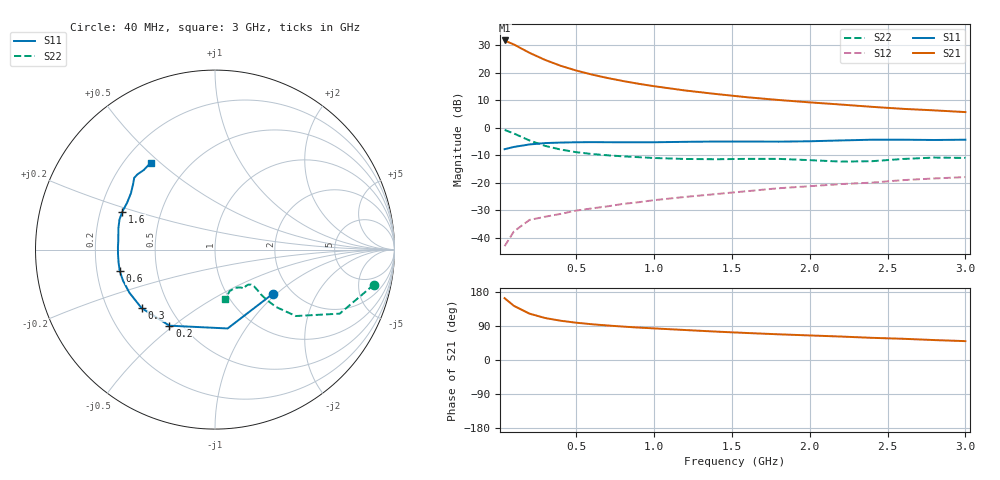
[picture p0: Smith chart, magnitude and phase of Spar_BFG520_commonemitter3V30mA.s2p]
! Filename:  BFG520F.S2P  Version:  2.1
! NXP part #: BFG520  Date: Feb 1992
! Bias condition: Vce=3V, Ic=30mA
! IN LINE PINNING: same data as with cross emitter pinning.
#  MHz  S  MA  R  50
! Freq  S11  S21  S12  S22  !GUM [dB]
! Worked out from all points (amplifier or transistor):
!   21 points, 40 MHz to 3 GHz, reference 50 ohm
!   highest |S21| = 31.7 dB at 40 MHz (marker M1)
!   |S21| within 3 dB of that: start of sweep to 150.3 MHz
!   unconditionally stable (mu >= 1): 627.5 MHz to end of sweep
!   at 300 MHz: K = 0.67, MSG = 28.5 dB, |S12| = -32.4 dB
!   at 1 GHz: K = 1.19, MAG = 18.1 dB, |S12| = -26.4 dB
!   at 3 GHz: K = 1.29, MAG = 8.6 dB, |S12| = -18.0 dB
!   S11 on the Smith chart (normalised r, x): 40 MHz: 1.60, -0.95; 200 MHz: 0.43, -0.48; 300 MHz: 0.35, -0.31; 600 MHz: 0.30, -0.10; 1.6 GHz: 0.29, +0.18; 3 GHz: 0.31, +0.47
40  0.405 -37.6  38.3 163.1  0.007 75.3  0.907 -12.4
100  0.445 -80.9  32.27 142.8  0.013 64.8  0.781 -27.2
200  0.494 -120.9  22.82 122.3  0.021 54.9  0.583 -39.4
300  0.523 -141.4  16.96 110.8  0.024 52.4  0.465 -43.3
400  0.534 -153.3  13.27 103.6  0.027 54.0  0.399 -44.2
500  0.541 -161.4  10.88 98.4  0.031 55.0  0.357 -44.3
600  0.544 -167.4  9.206 94.4  0.034 57.2  0.331 -43.7
700  0.542 -172.3  7.97 91.1  0.037 59.0  0.314 -43.5
800  0.541 -177.1  7.019 88.2  0.041 61.1  0.3 -43.2
900  0.541 178.5  6.255 85.6  0.044 63.2  0.29 -43.4
1000  0.541 174.6  5.65 83.4  0.048 64.8  0.28 -44.1
1200  0.551 167.7  4.721 79.1  0.055 66.4  0.269 -46.6
1400  0.558 162.5  4.07 74.9  0.062 67.7  0.266 -50.1
1600  0.558 157.8  3.553 71.2  0.07 69.7  0.27 -52.3
1800  0.555 152.0  3.172 67.8  0.079 69.5  0.27 -53.4
2000  0.564 146.1  2.871 64.8  0.086 70.9  0.256 -55.5
2200  0.584 141.4  2.622 61.9  0.094 71.0  0.241 -61.8
2400  0.602 138.4  2.383 58.5  0.1 72.0  0.245 -70.4
2600  0.602 135.8  2.189 56.0  0.111 71.6  0.269 -76.2
2800  0.595 131.8  2.055 52.6  0.119 69.8  0.285 -77.6
3000  0.602 126.5  1.912 49.8  0.126 70.8  0.281 -78.9
